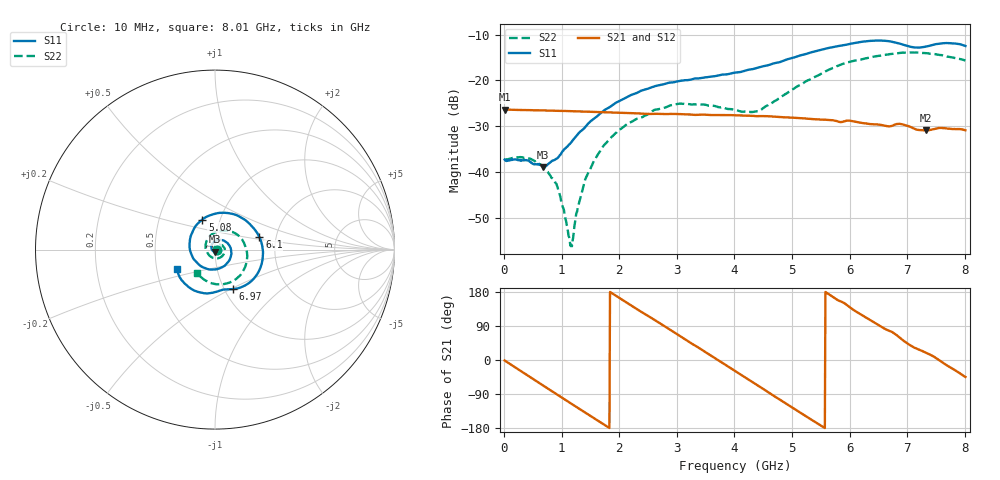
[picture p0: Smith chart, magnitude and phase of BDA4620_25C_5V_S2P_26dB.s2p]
!Agilent Technologies,E5071B,MY42404982,A.09.10
!Date: Wed May 06 09:04:05 2026
!Data & Calibration Information:
!Freq	S11:SOLT2(ON)	S21:SOLT2(ON)	S12:SOLT2(ON)	S22:SOLT2(ON)
# Hz S RI R 50
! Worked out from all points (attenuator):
!   801 points, 10 MHz to 8.01 GHz, reference 50 ohm
!   highest |S21| = -26.38 dB at 20 MHz (marker M1); lowest = -31.0 dB at 7.32 GHz (marker M2)
!   lowest |S11| = -38.9 dB at 680 MHz (marker M3), VSWR 1.02, Z = 49.8 - j1.11 ohm
!   |S11| at or under -10 dB: start of sweep to end of sweep
!   |S22| runs from -56.2 to -13.9 dB; largest |S21 - S12| = 0.00026
!   S11 on the Smith chart (normalised r, x): 10 MHz: 1.03, -0.00; 5.08 GHz: 0.82, +0.28; 6.1 GHz: 1.64, +0.24; 6.97 GHz: 1.09, -0.51; 8.01 GHz: 0.64, -0.14
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1e7  0.0136 -0.000881  0.0479 -0.000989  0.048 -0.000982  0.0135 -0.000429
2e7  0.0133 -0.000954  0.0479 -0.00177  0.048 -0.00195  0.0136 -0.000331
4.3e8  0.00792 -0.0106  0.0347 -0.0321  0.0347 -0.0322  0.0132 -0.00482
6.8e8  -0.00184 -0.0112  0.018 -0.0433  0.018 -0.0434  0.0092 -0.00651
9.3e8  -0.0131 -0.00526  -0.00155 -0.0465  -0.00167 -0.0465  0.00359 -0.00577
1.16e9  -0.0195 0.00724  -0.019 -0.0419  -0.0191 -0.042  -0.00134 -0.000769
1.35e9  -0.0199 0.0204  -0.0311 -0.0334  -0.0312 -0.0334  -0.00328 0.0049
1.53e9  -0.0145 0.0338  -0.0394 -0.0224  -0.0394 -0.0224  -0.00301 0.0115
1.77e9  0.00138 0.0483  -0.0446 -0.00494  -0.0446 -0.00493  0.0011 0.0205
2.14e9  0.0397 0.0526  -0.0384 0.0217  -0.0384 0.0218  0.0168 0.0289
2.68e9  0.088 0.00607  -0.00693 0.0424  -0.00687 0.0425  0.0444 0.0192
3.08e9  0.0819 -0.056  0.0208 0.0373  0.021 0.0373  0.055 -0.00758
4.01e9  -0.0798 -0.0911  0.0363 -0.02  0.0364 -0.0201  -0.0106 -0.0463
4.43e9  -0.1389 -0.00395  0.0143 -0.038  0.0143 -0.0381  -0.045 -0.0115
5.08e9  -0.0707 0.1672  -0.0263 -0.0285  -0.0264 -0.0285  -0.0212 0.0825
5.35e9  0.014 0.2031  -0.0352 -0.0136  -0.0353 -0.0137  0.0231 0.1023
6.1e9  0.2478 0.0687  -0.0221 0.0274  -0.0222 0.0274  0.1595 0.0414
6.68e9  0.2017 -0.1764  0.00681 0.0306  0.00685 0.0306  0.1696 -0.0898
6.97e9  0.0981 -0.2203  0.0219 0.0237  0.022 0.0238  0.1306 -0.1526
7.32e9  0.0131 -0.2334  0.0267 0.00946  0.0268 0.00946  0.0489 -0.1924
7.65e9  -0.1114 -0.2298  0.0295 -0.00528  0.0295 -0.00533  -0.0326 -0.1829
8.01e9  -0.2121 -0.1067  0.0202 -0.02  0.0202 -0.0201  -0.1028 -0.1283
